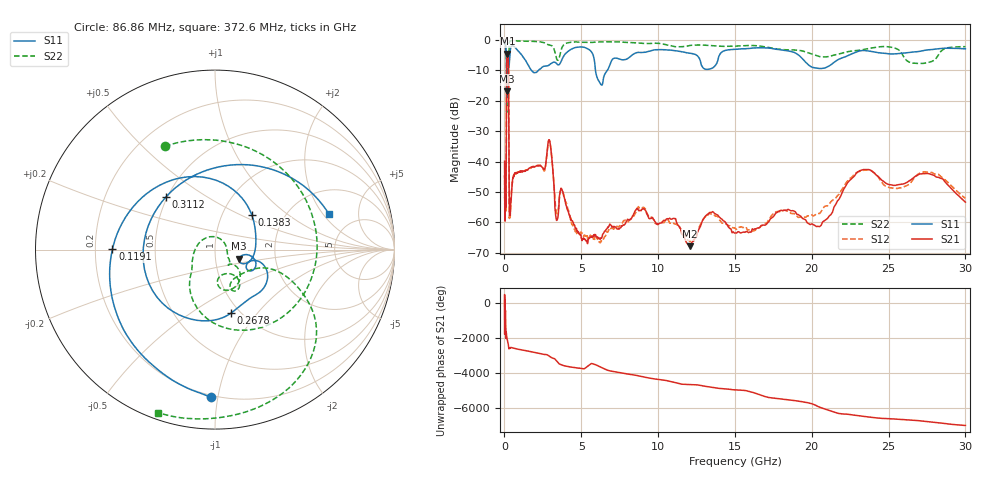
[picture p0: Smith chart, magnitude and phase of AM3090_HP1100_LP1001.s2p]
! Date/Time: Thu, Feb 28, 2019 2:06 PM
! Network Analyzer: Agilent Technologies E8364B Rev: A.07.50.67
! Sweep from 0.010 to 30.000 GHz, 1601 Points, Sweep Type: LOG
! Power Supply: 5.023 V, 0.002 A
# Hz S DB R 50
!freq MagS11 AngS11 MagS21 AngS21 MagS12 AngS12 MagS22 AngS22
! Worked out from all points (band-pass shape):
!   1601 points, 10 MHz to 30 GHz, reference 50 ohm
!   highest |S21| = -4.46 dB at 188.7 MHz (marker M1); lowest = -67.8 dB at 12.07 GHz (marker M2)
!   |S21| within 3 dB of the highest: 142.5 MHz to 253.9 MHz (111.4 MHz wide, 56.2 % of centre)
!   lowest |S11| = -16.8 dB at 166.5 MHz (marker M3), VSWR 1.34, Z = 65.1 - j6.81 ohm
!   |S11| at or under -10 dB: 136.1 MHz to 230.9 MHz (94.84 MHz wide, 51.7 % of centre); 1.763 GHz to 2.202 GHz (438.8 MHz wide, 22.1 % of centre); 5.925 GHz to 6.694 GHz (768.6 MHz wide, 12.2 % of centre)
!   |S22| runs from -23.8 to -0.1 dB; largest |S21 - S12| = 0.015
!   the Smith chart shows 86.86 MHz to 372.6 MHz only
!   S11 on the Smith chart (normalised r, x): 86.86 MHz: 0.19, -0.95; 119.1 MHz: 0.27, +0.00; 138.3 MHz: 1.37, +0.58; 267.8 MHz: 0.91, -0.74; 311.2 MHz: 0.49, +0.34; 372.6 MHz: 3.20, +2.30
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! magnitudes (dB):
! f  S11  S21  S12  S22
! 10 MHz  -0.2  -39.8  -45.6  -0.6
! 38.04 MHz  -0.4  -55.9  -56.8  -1.4
! 86.86 MHz  -1.7  -52.1  -54.2  -3.9
! 105.6 MHz  -3.1  -52.4  -54.4  -4.7
! 119.1 MHz  -4.9  -36.2  -36.4  -5.2
! 138.3 MHz  -11.0  -9.5  -9.4  -21.7
! 144.7 MHz  -12.6  -6.8  -6.8  -23.4
! 166.5 MHz  -16.8  -4.7  -4.7  -17.4
! 188.7 MHz  -12.3  -4.5  -4.4  -12.4
! 267.8 MHz  -8.8  -11.9  -11.9  -10.8
! 311.2 MHz  -7.9  -53.8  -55.6  -0.9
! 372.6 MHz  -3.5  -57.8  -58.2  -0.3
! 550.5 MHz  -1.9  -45.3  -45.5  -0.2
! 2.084 GHz  -10.6  -41.4  -41.2  -0.5
! 2.913 GHz  -8.2  -32.9  -32.8  -1.6
! 3.402 GHz  -7.8  -59.3  -57.0  -6.3
! 3.723 GHz  -6.6  -49.0  -49.1  -2.8
! 7.926 GHz  -6.3  -59.7  -59.6  -0.8
! 12.07 GHz  -4.3  -67.8  -66.3  -1.8
! 20.51 GHz  -9.4  -61.4  -57.1  -5.4
! 23.36 GHz  -3.4  -42.6  -42.9  -3.1
! 30 GHz  -2.9  -53.3  -52.0  -2.2
